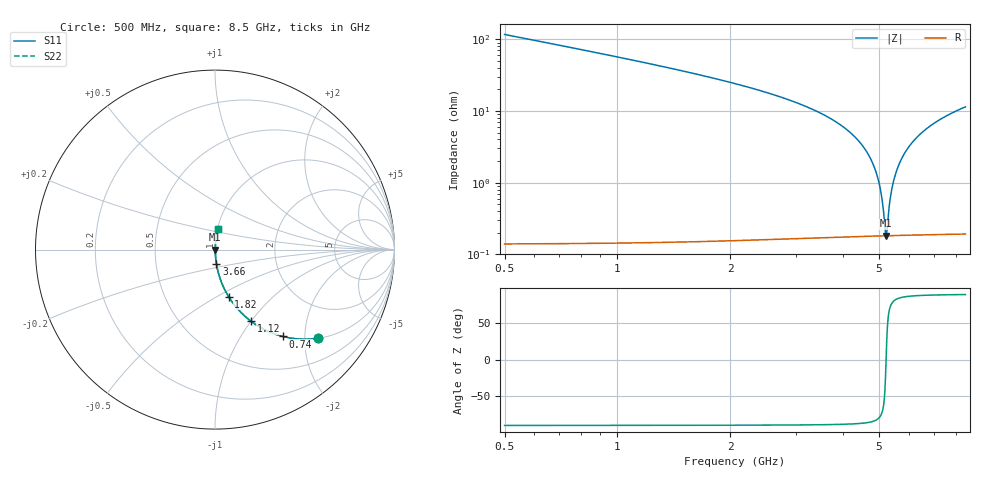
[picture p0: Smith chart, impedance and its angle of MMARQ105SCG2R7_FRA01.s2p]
! MMARQ105SCG2R7_FRA01  S-PARAMETER MODEL  ( General Type )
! Model Generated by TAIYO YUDEN Corporation (http://www.ty-top.com)
! Version 1.0
! TAIYO YUDEN Control No. 200326
! Copyright(c) 2020 TAIYO YUDEN CO.,LTD. All Rights Reserved.
! Product Description (link to TY-COMPAS)
! https://ds.yuden.co.jp/TYCOMPAS/or/detail?pn=MMARQ105SCG2R7BFRA01&u=M
! Products Name : Multilayer Ceramic Capacitors
! Characteristics :
!  Capacitance : 2.7 pF , Rated Voltage : 250V , TCC : CG / C0G
!  Case Size : 1.0 x 0.5 / 0.039 x 0.02 [mm/inch] , Thickness : 0.5 / 0.02 [mm/inch]
!  (Conditions: Temperature = 25 degC , DC Bias Current/Voltage = 0A / 0V)
! External Node Assignments :
!  1  o---| |---o  2
! GND o---------o GND
! Frequency Range : 500MHz  -  8.5GHz  [ 401 STEP ]
# MHz S RI R 50
! Freq[MHz].  S11 Real  S11 Imag  S21 Real  S21 Imag  S12 Real  S12 Imag  S22 Real  S22 Imag
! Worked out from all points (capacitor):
!   401 points, 500 MHz to 8.5 GHz, reference 50 ohm
!   read as one part in series: C = 2.71 pF near 540 MHz
!   lowest |Z| = 182 mohm at 5.22 GHz (marker M1)
!   series resonance near 5.22 GHz, so ESL is about 340 pH
!   S11 on the Smith chart (normalised r, x): 500 MHz: 1.00, -2.33; 740 MHz: 1.00, -1.56; 1.12 GHz: 1.00, -1.00; 1.82 GHz: 1.00, -0.57; 3.66 GHz: 1.00, -0.16; 8.5 GHz: 1.00, +0.23
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500  0.5759 -0.4936  0.4241 0.4936  0.4241 0.4936  0.5759 -0.4936
740  0.3777 -0.4839  0.6223 0.4839  0.6223 0.4839  0.3777 -0.4839
1120  0.2012 -0.3995  0.7988 0.3995  0.7988 0.3995  0.2012 -0.3995
1820  0.0757 -0.2618  0.9243 0.2618  0.9243 0.2618  0.0757 -0.2618
1840  0.0738 -0.2587  0.9262 0.2587  0.9262 0.2587  0.0738 -0.2587
3180  0.0149 -0.1143  0.9851 0.1143  0.9851 0.1143  0.0149 -0.1143
3660  0.00829 -0.0808  0.9917 0.0808  0.9917 0.0808  0.00829 -0.0808
4140  0.0045 -0.0523  0.9955 0.0523  0.9955 0.0523  0.0045 -0.0523
4500  0.00289 -0.0334  0.9971 0.0334  0.9971 0.0334  0.00289 -0.0334
4760  0.00222 -0.0207  0.9978 0.0207  0.9978 0.0207  0.00222 -0.0207
4960  0.00193 -0.0115  0.9981 0.0115  0.9981 0.0115  0.00193 -0.0115
5080  0.00184 -0.00609  0.9982 0.00609  0.9982 0.00609  0.00184 -0.00609
5180  0.00182 -0.00172  0.9982 0.00172  0.9982 0.00172  0.00182 -0.00172
5220  0.00181 3.98e-06  0.9982 -3.98e-06  0.9982 -3.98e-06  0.00181 3.98e-06
5260  0.00182 0.00172  0.9982 -0.00172  0.9982 -0.00172  0.00182 0.00172
5360  0.00186 0.00594  0.9981 -0.00594  0.9981 -0.00594  0.00186 0.00594
5460  0.00193 0.0101  0.9981 -0.0101  0.9981 -0.0101  0.00193 0.0101
5620  0.00211 0.0166  0.9979 -0.0166  0.9979 -0.0166  0.00211 0.0166
5840  0.00248 0.0252  0.9975 -0.0252  0.9975 -0.0252  0.00248 0.0252
6380  0.00391 0.0452  0.9961 -0.0452  0.9961 -0.0452  0.00391 0.0452
7180  0.00715 0.0723  0.9929 -0.0723  0.9929 -0.0723  0.00715 0.0723
8500  0.0147 0.1122  0.9853 -0.1122  0.9853 -0.1122  0.0147 0.1122
